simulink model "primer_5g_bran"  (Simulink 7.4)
settings: Solver=FixedStepDiscrete  StartTime=0.0  StopTime=5e-6  RelTol=1e-3
undefined symbols (not defined in the file or in its folder): interp1
libraries: powerlib x11

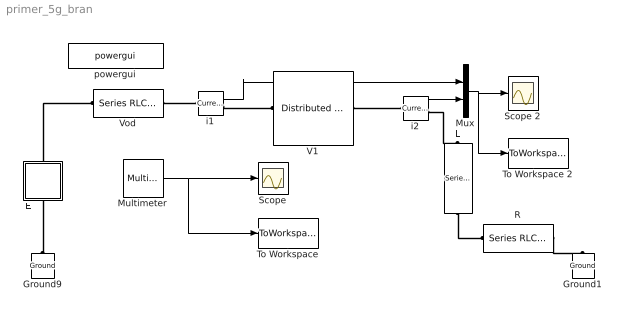
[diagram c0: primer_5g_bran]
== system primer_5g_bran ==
  E : Subsystem  mask(Proizvolen generator){vreme=[0 0.001 0.5 0.501 50]/1e6, napon=2*[0 500 500 0 0]*1000}
      mask prompts: vreme "Vreme (s)"; napon "Napon (V)"
      mask help: So ovoj element e definiran idealen naponski generator so proizvolen oblik. Oblikot na naponot se definira so pomos na dva vektori, pri sto vo prviot vektor se dadeni diskretni vremenski momenti dodeka vrednostite na naponot vo tie momenti se dadeni vo vtoriot vektor. Za ostanatite vremenski momenti koi sto ne se dadeni vo vektorite modelot pravi linearna interpolacija.
  Ground1 : powerlib/Elements/Ground  DialogController=POWERSYS.PowerSysDialog  PhysicalDomain=powersysdomain  SubClassName=unknown  LeftPortType=p1  RightPortType=p1  LConnTagsString=a
  Ground9 : powerlib/Elements/Ground  DialogController=POWERSYS.PowerSysDialog  PhysicalDomain=powersysdomain  SubClassName=unknown  LeftPortType=p1  RightPortType=p1  LConnTagsString=a
  L : powerlib/Elements/Series RLC Branch  DialogController=POWERSYS.PowerSysDialog  PhysicalDomain=powersysdomain  SubClassName=unknown  LeftPortType=p1  RightPortType=p1  LConnTagsString=__new0  RConnTagsString=__new0  BranchType=L  Resistance=400  Inductance=1e-3  SetiL0=on  InitialCurrent=0  Capacitance=5e-9  Setx0=on  InitialVoltage=0  Measurements=None
  Multimeter : powerlib/Measurements/Multimeter  SystemSampleTime=-1  PhasorSimulation=off  OutputType=Complex  sel=[1 2]  L=3  Gain=[1 1]  yselected={'Us_ph1_gnd: V1','Ur_ph1_gnd: V1'};  PSBOutputType=1  PSBequivalent=0  AxesSetting=[0,0.1,-100,100]  Display=0  SavedBlockNames=-11
  Mux : Mux  Inputs=2
  R : powerlib/Elements/Series RLC Branch  DialogController=POWERSYS.PowerSysDialog  PhysicalDomain=powersysdomain  SubClassName=unknown  LeftPortType=p1  RightPortType=p1  LConnTagsString=__new0  RConnTagsString=__new0  BranchType=R  Resistance=400  Inductance=1e-3  SetiL0=on  InitialCurrent=0  Capacitance=5e-9  Setx0=on  InitialVoltage=0  Measurements=None
  Scope : Scope
  Scope 2 : Scope
  To Workspace : ToWorkspace  VariableName=naponi  SampleTime=-1  SaveFormat=Structure With Time
  To Workspace 2 : ToWorkspace  VariableName=strui  SampleTime=-1  SaveFormat=Structure With Time
  V1 : powerlib/Elements/Distributed Parameters Line  DialogController=POWERSYS.PowerSysDialog  SystemSampleTime=-1  Phases=1  Frequency=50  Resistance=0.001  Inductance=1.334e-3  Capacitance=8.334e-009  Length=0.3  x1=[0 0;2.00057995591278e-007 0;4.00115991182557e-007 0;6.00173986773835e-007 0;8.00231982365114e-007 0;1.00028997795639e-006 0]  x2=[0 0;2.00057995591278e-007 0;4.00115991182557e-007 0;6.00173986773835e-007 0;8.00231982365114e-007 0;1.00028997795639e-006 0]  x3=[0 0;2.00057995591278e-007 0;4.00115991182557e-007 0;6.00173986773835e-007 0;8.00231982365114e-007 0;1.00028997795639e-006 0]  x4=[0 0;2.00057995591278e-007 0;4.00115991182557e-007 0;6.00173986773835e-007 0;8.00231982365114e-007 0;1.00028997795639e-006 0]  x5=1.00028997795639e-006  Measurements=Phase-to-ground voltages
  Vod : powerlib/Elements/Series RLC Branch  DialogController=POWERSYS.PowerSysDialog  PhysicalDomain=powersysdomain  SubClassName=unknown  LeftPortType=p1  RightPortType=p1  LConnTagsString=__new0  RConnTagsString=__new0  BranchType=R  Resistance=400  Inductance=1e-3  SetiL0=off  InitialCurrent=0  Capacitance=1e-6  Setx0=off  InitialVoltage=0  Measurements=None
  i1 : powerlib/Measurements/Current Measurement  DialogController=POWERSYS.PowerSysDialog  SystemSampleTime=-1  PhasorSimulation=off  OutputType=Complex  PSBequivalent=0
  i2 : powerlib/Measurements/Current Measurement  DialogController=POWERSYS.PowerSysDialog  SystemSampleTime=-1  PhasorSimulation=off  OutputType=Complex  PSBequivalent=0
  powergui : powerlib/powergui  SystemSampleTime=-1  SimulationMode=Discrete  SampleTime=1e-8  frequency=60  SPID=off  DisableSnubberDevices=off  DisableRonSwitches=off  DisableVfSwitches=off  SwTol=0  Interpol=off  frequencyindice=0  echomessages=off  HookPort=off  DisplayEquations=off  FunctionMessages=off  EnableUseOfTLC=off  x0status=blocks  RestoreLinks=warning  Frange=[0:2:500]  Ylog=off  Xlog=on  ShowGrid=off  save=off  variable=ZData  ZoomFFT=on  StartTime=0.0  cycles=1  DisplayStyle=1  fundamental=60  FreqAxis=off  MaxFrequency=1000  frequencyindicesteady=1  RmsSteady=1  display=off  Ts=0  methode=off
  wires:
  Multimeter/1 -> Scope/1, To Workspace/1
  i1/1 -> Mux/1
  i2/1 -> Mux/2
  Mux/1 -> Scope 2/1, To Workspace 2/1
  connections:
  Ground9/LConn1 -- E/LConn1
  E/RConn1 -- Vod/LConn1
  Vod/RConn1 -- i1/LConn1
  i1/RConn1 -- V1/LConn1
  V1/RConn1 -- i2/LConn1
  i2/RConn1 -- L/LConn1
  L/RConn1 -- R/RConn1
  R/LConn1 -- Ground1/LConn1

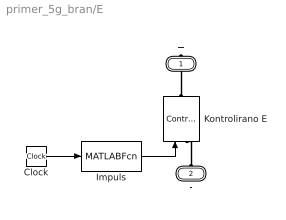
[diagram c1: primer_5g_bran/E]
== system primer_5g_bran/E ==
  Clock : Clock
  Impuls : MATLABFcn  MATLABFcn=interp1(vreme, napon, u)  OutputSignalType=real
  Kontrolirano E : powerlib/Electrical Sources/Controlled Voltage Source  DialogController=POWERSYS.PowerSysDialog  SystemSampleTime=-1  Initialize=on  Source_Type=AC  Amplitude=0  Phase=0  Frequency=0  Measurements=Voltage
  + : PMIOPort  Port=1  Side=Right
  - : PMIOPort  Port=2  Side=Left
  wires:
  Impuls/1 -> Kontrolirano E/1
  Clock/1 -> Impuls/1
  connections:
  +/RConn1 -- Kontrolirano E/RConn1
  -/RConn1 -- Kontrolirano E/LConn1
